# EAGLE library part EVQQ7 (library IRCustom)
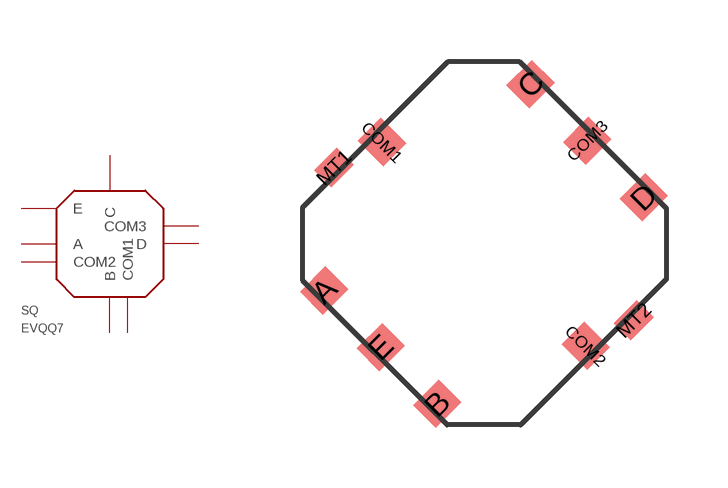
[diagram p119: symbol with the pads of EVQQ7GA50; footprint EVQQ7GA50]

Designator prefix SQ

## EVQQ7GA50  [EVQQ7GA50]
A  A
B  B
C  C
COM1  COM1
COM2  COM2
COM3  COM3
D  D
E  E

## Footprint EVQQ7GA50 (pad centres in mm)
smd 0.8 x 0.9 rotated 135: A -3.995,-1.167; B -1.167,-3.995; C 1.167,3.995; COM3 2.581,2.581; D 3.995,1.167; E -2.581,-2.581
smd 0.8 x 0.9 rotated 45: COM1 -2.546,2.546; COM2 2.546,-2.546
smd 0.8 x 0.6 rotated 45: MT1 -3.748,1.909; MT2 3.748,-1.909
